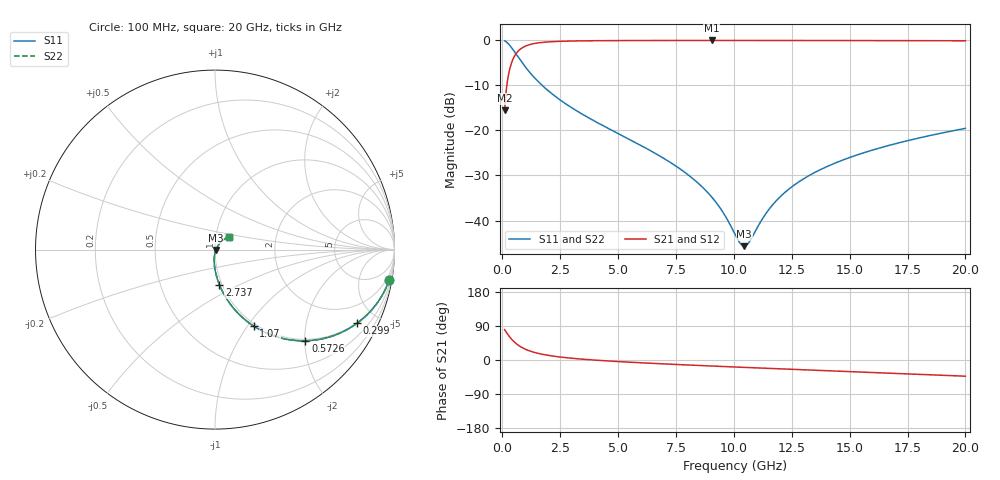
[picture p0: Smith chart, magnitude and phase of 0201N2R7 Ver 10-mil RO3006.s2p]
# GHz S MA R 50
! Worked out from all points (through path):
!   1601 points, 100 MHz to 20 GHz, reference 50 ohm
!   highest |S21| = -0.05 dB at 9.043 GHz (marker M1); lowest = -15.5 dB at 100 MHz (marker M2)
!   group delay of S21, straight-line fit = 9.51 ps
!   lowest |S11| = -45.7 dB at 10.45 GHz (marker M3), VSWR 1.01, Z = 50.5 - j0.185 ohm
!   |S11| at or under -10 dB: 1.72 GHz to end of sweep
!   |S22| runs from -45.7 to -0.1 dB; largest |S21 - S12| = 0
!   S11 on the Smith chart (normalised r, x): 100 MHz: 1, -12; 299 MHz: 0.97, -3.86; 572.6 MHz: 0.97, -2.01; 1.07 GHz: 0.97, -1.07; 2.737 GHz: 0.97, -0.40; 20 GHz: 1.15, +0.17
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0.1  0.9858 -9.8  0.1673 80.2  0.1673 80.2  0.9858 -9.8
0.299  0.8912 -27.5  0.4525 62.5  0.4525 62.5  0.8912 -27.5
0.423375  0.8111 -36.5  0.5835 53.4  0.5835 53.4  0.8111 -36.5
0.572625  0.7154 -45.3  0.697 44.6  0.697 44.6  0.7154 -45.3
0.8089375  0.5858 -55.5  0.8084 34.3  0.8084 34.3  0.5858 -55.5
1.070125  0.4779 -63.2  0.876 26.5  0.876 26.5  0.4779 -63.2
1.704438  0.3189 -74.1  0.9449 15.4  0.9449 15.4  0.3189 -74.1
2.73675  0.1974 -82.8  0.977 6.2  0.977 6.2  0.1974 -82.8
3.420812  0.1532 -86.3  0.9846 2.4  0.9846 2.4  0.1532 -86.3
6.741625  0.0531 -94.8  0.994 -9.6  0.994 -9.6  0.0531 -94.8
8.072437  0.03146 -94.7  0.9946 -13.3  0.9946 -13.3  0.03146 -94.7
9.042563  0.01825 -90.3  0.9947 -15.9  0.9947 -15.9  0.01825 -90.3
9.5525  0.0121 -82.7  0.9947 -17.2  0.9947 -17.2  0.0121 -82.7
10.05  0.007059 -62.0  0.9946 -18.5  0.9946 -18.5  0.007059 -62.0
10.448  0.005198 -20.6  0.9945 -19.5  0.9945 -19.5  0.005198 -20.6
10.65944  0.005753 4.4  0.9945 -20.0  0.9945 -20.0  0.005753 4.4
11.30619  0.01116 39.6  0.9943 -21.7  0.9943 -21.7  0.01116 39.6
11.85344  0.01681 48.0  0.9941 -23.0  0.9941 -23.0  0.01681 48.0
13.37081  0.03284 53.2  0.9934 -26.7  0.9934 -26.7  0.03284 53.2
14.81356  0.04805 52.6  0.9925 -30.2  0.9925 -30.2  0.04805 52.6
16.69162  0.06808 49.9  0.9909 -34.7  0.9909 -34.7  0.06808 49.9
20  0.1053 43.5  0.987 -42.7  0.987 -42.7  0.1053 43.5
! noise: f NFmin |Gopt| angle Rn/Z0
0.1  0.0009547  0.9553  0.5477  0.00481
2.301  0.005357  0.8259  4.59  0.006457
4.515  0.008287  0.7845  8.672  0.007854
6.729  0.01081  0.7581  12.74  0.008938
8.943  0.01312  0.739  16.79  0.009854
11.14  0.01528  0.7245  20.77  0.01066
13.36  0.01736  0.713  24.73  0.0114
15.57  0.01938  0.7039  28.63  0.01208
17.79  0.02136  0.6968  32.48  0.01272
20  0.02332  0.6912  36.27  0.01333
